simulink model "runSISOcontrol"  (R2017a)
settings: Solver=VariableStepAuto  StartTime=0.0  StopTime=12  RelTol=1e-3
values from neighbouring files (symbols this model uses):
  baud = 250000    [MISOcontrol.m]    (also in MISO_demo.m; runSteptest.m; SISOcontrol.m; init.m)
  com = 'COM4'    [MISOcontrol.m]    (also in MISO_demo.m; runSteptest.m; SISOcontrol.m; init.m)
  fixed_u1 = 0    [MISOcontrol.m]    (also in MISO_demo.m; SISOcontrol.m; init.m)
  fixed_u2 = 0    [MISOcontrol.m]    (also in MISO_demo.m; SISOcontrol.m; init.m)
  fixed_u3 = 0    [MISOcontrol.m]    (also in MISO_demo.m; SISOcontrol.m; init.m)
  fTf = 0.1    [MISOcontrol.m]    (also in MISO_demo.m; runSteptest.m; SISOcontrol.m; init.m)
  fTl = 0.05    [MISOcontrol.m]    (also in MISO_demo.m; runSteptest.m; SISOcontrol.m; init.m)
  fTt = 0.05    [MISOcontrol.m]    (also in MISO_demo.m; runSteptest.m; SISOcontrol.m; init.m)
  Kc = 1/k*tau1/(tauc+theta)    [SIMCPI.m]    (also in SIMCPI_nosat.m)
  step_d1 = -2.5    [MISOcontrol.m]    (also in MISO_demo.m; SISOcontrol.m = -2; init.m = 0)
  step_d2 = +2.5    (= 2.5)    [MISOcontrol.m]    (also in MISO_demo.m; SISOcontrol.m = 2; init.m = 0)
  step_ys1 = 5    [MISOcontrol.m]    (also in MISO_demo.m; SISOcontrol.m = 4)
  step_ys2 = -5    [MISOcontrol.m]    (also in MISO_demo.m; SISOcontrol.m = -4)
  stepTime1 = 30    [MISO_demo.m]    (also in SISOcontrol.m = 2)
  stepTime2 = 60    [MISO_demo.m]    (also in SISOcontrol.m = 4)
  stepTime_d1 = 90    [MISOcontrol.m]    (also in MISO_demo.m; SISOcontrol.m = 6; init.m = 0)
  stepTime_d2 = 120    [MISOcontrol.m]    (also in MISO_demo.m; SISOcontrol.m = 8; init.m = 0)
  tauI = min(tau1,4*(tauc+theta))    [SIMCPI.m]    (also in SIMCPI_nosat.m)
  Ts = 0.1    [identification.m]    (also in MISOcontrol.m; MISO_demo.m; runSteptest.m; SISOcontrol.m)
  turnOn_u1 = 1    [MISOcontrol.m]    (also in MISO_demo.m; SISOcontrol.m = 0)
  turnOn_u2 = 1    [MISOcontrol.m]    (also in MISO_demo.m; SISOcontrol.m = 0)
  turnOn_u3 = 0    [MISOcontrol.m]    (also in MISO_demo.m; SISOcontrol.m = 1)
  turnOn_y1 = 1    [MISOcontrol.m]    (also in MISO_demo.m; SISOcontrol.m = 0)
  turnOn_y2 = 0    [MISOcontrol.m]    (also in MISO_demo.m; SISOcontrol.m = 1)
  y0 = sb_T+3    (= 30)    [MISOcontrol.m]    (also in MISO_demo.m = sb_T; SISOcontrol.m = 0; init.m = 0; MIMOcontrol.m = 27)
  y_s0 = 0    [MISOcontrol.m]    (also in MISO_demo.m; SISOcontrol.m = 4)
undefined symbols (not defined in the file or in its folder): Kb
libraries: simulink x1, tom_lib x1

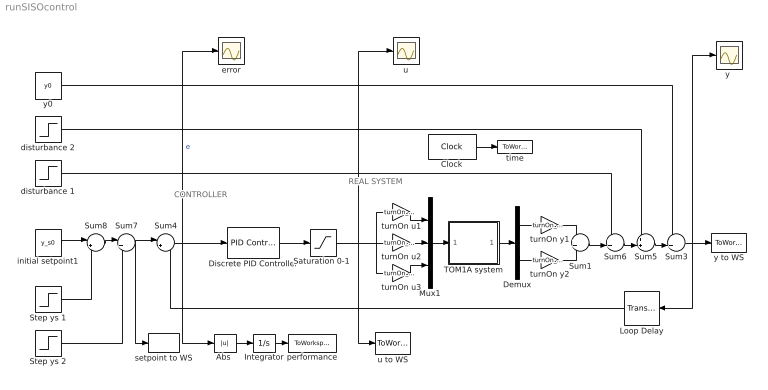
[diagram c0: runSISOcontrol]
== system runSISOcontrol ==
  note: CONTROLLER
  note: REAL SYSTEM
  "Abs " : Abs  ZeroCross=off
  Clock : Clock
  Demux : Demux  Outputs=2
  Discrete PID Controller : simulink/Continuous/PID Controller  Controller=PI  TimeDomain=Discrete-time  SampleTime=Ts  IntegratorMethod=Forward Euler  FilterMethod=Forward Euler  Form=Parallel  UseFilter=on  ControllerParametersSource=internal  P=Kc  I=Kc/tauI  D=0  N=100  InitialConditionSource=internal  InitialConditionForIntegrator=0  InitialConditionForFilter=0  ExternalReset=none  ZeroCross=off  LimitOutput=on  UpperSaturationLimit=1  LowerSaturationLimit=0  LinearizeAsGain=off  AntiWindupMode=clamping  Kb=Kb  TrackingMode=off  Kt=1  PParamMin=[]  PParamMax=[]  IParamMin=[]  IParamMax=[]  DParamMin=[]  DParamMax=[]  NParamMin=[]  NParamMax=[]  KbParamMin=[]  KbParamMax=[]  KtParamMin=[]  KtParamMax=[]  POutMin=[]  POutMax=[]  IOutMin=[]  IOutMax=[]  DOutMin=[]  DOutMax=[]  NOutMin=[]  NOutMax=[]  KbOutMin=[]  KbOutMax=[]  KtOutMin=[]  KtOutMax=[]  IntegratorOutMin=[]  IntegratorOutMax=[]  FilterOutMin=[]  FilterOutMax=[]  SumOutMin=[]  SumOutMax=[]  SumI1OutMin=[]  SumI1OutMax=[]  SumI2OutMin=[]  SumI2OutMax=[]  SumI3OutMin=[]  SumI3OutMax=[]  SumDOutMin=[]  SumDOutMax=[]  SaturationOutMin=[]  SaturationOutMax=[]  IntegratorContinuousStateAttributes=''  IntegratorStateMustResolveToSignalObject=off  IntegratorRTWStateStorageClass=Auto  FilterContinuousStateAttributes=''  FilterStateMustResolveToSignalObject=off  FilterRTWStateStorageClass=Auto  DifferentiatorICPrevScaledInput=0  DifferentiatorOutMin=[]  DifferentiatorOutMax=[]  InitialConditionSetting=State (most efficient)
  Integrator : Integrator  ZeroCross=off
  Loop Delay : TransportDelay  DelayTime=0.1
  Mux1 : Mux  Inputs=3
  "Saturation 0-1 " : Saturate  UpperLimit=1  LowerLimit=0  ZeroCross=off
  Step ys 1 : Step  Time=stepTime1  After=step_ys1  SampleTime=Ts  ZeroCross=off
  Step ys 2 : Step  Time=stepTime2  After=step_ys2  SampleTime=Ts  ZeroCross=off
  Sum1 : Sum
  Sum3 : Sum  Inputs=-+|
  Sum4 : Sum  Inputs=|+-
  Sum5 : Sum  Inputs=++|
  Sum6 : Sum  Inputs=++|
  Sum7 : Sum  Inputs=|++
  Sum8 : Sum  Inputs=|++
  TOM1A system : Subsystem
  disturbance 1 : Step  Time=stepTime_d1  After=step_d1  SampleTime=Ts  ZeroCross=off
  disturbance 2 : Step  Time=stepTime_d2  After=step_d2  SampleTime=Ts  ZeroCross=off
  error : Scope
  initial setpoint1 : Constant  Value=y_s0  SampleTime=Ts
  performance : ToWorkspace  VariableName=IAE  SampleTime=Ts
  setpoint to WS : ToWorkspace  VariableName=ys  SampleTime=Ts
  time : ToWorkspace  VariableName=time  SampleTime=Ts
  turnOn u1 : Gain  Gain=turnOn_u1
  turnOn u2 : Gain  Gain=turnOn_u2
  turnOn u3 : Gain  Gain=turnOn_u3
  turnOn y1 : Gain  Gain=turnOn_y1
  turnOn y2 : Gain  Gain=turnOn_y2
  u : Scope
  u to WS : ToWorkspace  VariableName=u  SampleTime=-1
  "y " : Scope
  y to WS : ToWorkspace  VariableName=y  SampleTime=Ts
  y0 : Constant  Value=y0
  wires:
  Clock/1 -> time/1
  "Saturation 0-1 "/1 -> u/1, turnOn u3/1, turnOn u1/1, turnOn u2/1, u to WS/1
  disturbance 1/1 -> Sum6/1
  Sum3/1 -> y to WS/1, "y "/1, Loop Delay/1
  Sum7/1 -> setpoint to WS/1, Sum4/1
  "Abs "/1 -> Integrator/1
  TOM1A system/1(y) -> Demux/1
  Sum4/1 -> Discrete PID Controller/1, "Abs "/1, error/1  "e"
  Integrator/1 -> performance/1
  Mux1/1 -> TOM1A system/1(u)
  turnOn u1/1 -> Mux1/1
  turnOn u2/1 -> Mux1/2
  turnOn u3/1 -> Mux1/3
  Demux/1 -> turnOn y1/1
  Demux/2 -> turnOn y2/1
  turnOn y2/1 -> Sum1/2
  turnOn y1/1 -> Sum1/1
  Discrete PID Controller/1 -> "Saturation 0-1 "/1
  Loop Delay/1 -> Sum4/2
  Sum1/1 -> Sum6/2
  Sum6/1 -> Sum5/2
  disturbance 2/1 -> Sum5/1
  Sum5/1 -> Sum3/2
  y0/1 -> Sum3/1
  Step ys 2/1 -> Sum7/2
  Sum8/1 -> Sum7/1
  initial setpoint1/1 -> Sum8/1
  Step ys 1/1 -> Sum8/2

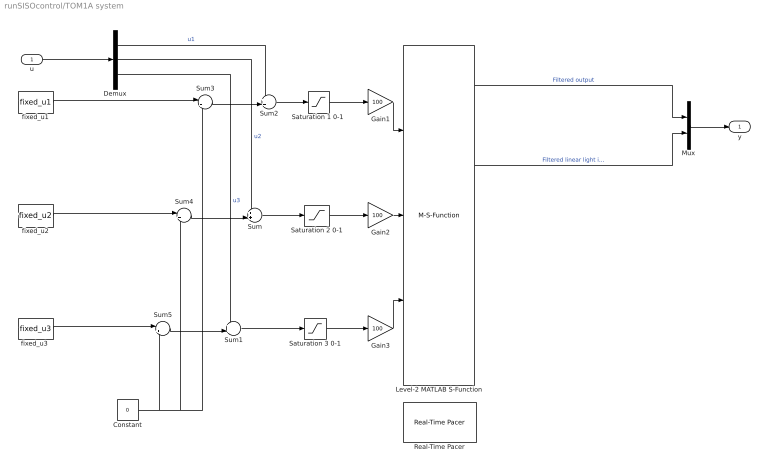
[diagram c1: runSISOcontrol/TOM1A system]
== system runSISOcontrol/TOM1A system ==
  u : Inport
  Constant : Constant  Value=0
  Demux : Demux  Outputs=3
  Gain1 : Gain  Gain=100
  Gain2 : Gain  Gain=100
  Gain3 : Gain  Gain=100
  Level-2 MATLAB S-Function : M-S-Function  FunctionName=tom1ar8  Parameters=Ts,com,baud,fTt,fTl,fTf
  Mux : Mux  Inputs=2
  Real-Time Pacer : tom_lib/Real-Time Pacer  simTimePerRealTime=1
  "Saturation 1 0-1 " : Saturate  UpperLimit=1  LowerLimit=0  ZeroCross=off
  Saturation 2 0-1 : Saturate  UpperLimit=1  LowerLimit=0  ZeroCross=off
  Saturation 3 0-1 : Saturate  UpperLimit=1  LowerLimit=0  ZeroCross=off
  Sum : Sum  Inputs=++|
  Sum1 : Sum  Inputs=++|
  Sum2 : Sum  Inputs=++|
  Sum3 : Sum  Inputs=|++
  Sum4 : Sum  Inputs=|++
  Sum5 : Sum  Inputs=|++
  fixed_u1 : Constant  Value=fixed_u1
  fixed_u2 : Constant  Value=fixed_u2
  "fixed_u3 " : Constant  Value=fixed_u3
  y : Outport
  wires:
  Level-2 MATLAB S-Function/14 -> ?  "Fan filtered  rpm"
  Level-2 MATLAB S-Function/3 -> ?  "Derivative of internal temperature"
  Level-2 MATLAB S-Function/4 -> ?  "Filtered external temperature"
  Level-2 MATLAB S-Function/13 -> ?  "Fan voltage"
  Level-2 MATLAB S-Function/11 -> ?  "Bulb voltage"
  Level-2 MATLAB S-Function/8 -> ?  "Filtered logaritmic light intensity"
  Level-2 MATLAB S-Function/1 -> ?  "Board temperature"
  Level-2 MATLAB S-Function/5 -> ?  "Derivate of external temperature"
  Level-2 MATLAB S-Function/12 -> ?  "Fan current"
  Level-2 MATLAB S-Function/9 -> ?  "Derivate of logaritmic light intensity"
  Level-2 MATLAB S-Function/16 -> ?  "Count of fan rpm"
  Level-2 MATLAB S-Function/15 -> ?  "Derivate of fan rpm"
  Level-2 MATLAB S-Function/10 -> ?  "Bulb current"
  Level-2 MATLAB S-Function/6 -> Mux/2  "Filtered linear light intensity"
  Level-2 MATLAB S-Function/7 -> ?  "Derivate of linear light intensity"
  Demux/1 -> Sum2/1  "u1"
  Demux/2 -> Sum/1  "u2"
  Demux/3 -> Sum1/1  "u3"
  u/1 -> Demux/1
  Level-2 MATLAB S-Function/2 -> Mux/1  "Filtered output"
  Mux/1 -> y/1
  fixed_u1/1 -> Sum3/1
  Sum3/1 -> Sum2/2
  Constant/1 -> Sum5/2, Sum4/2, Sum3/2
  fixed_u2/1 -> Sum4/1
  "fixed_u3 "/1 -> Sum5/1
  Sum5/1 -> Sum1/2
  Sum4/1 -> Sum/2
  Gain1/1 -> Level-2 MATLAB S-Function/1
  Gain2/1 -> Level-2 MATLAB S-Function/2
  Gain3/1 -> Level-2 MATLAB S-Function/3
  Saturation 2 0-1/1 -> Gain2/1
  Sum/1 -> Saturation 2 0-1/1
  "Saturation 1 0-1 "/1 -> Gain1/1
  Sum2/1 -> "Saturation 1 0-1 "/1
  Saturation 3 0-1/1 -> Gain3/1
  Sum1/1 -> Saturation 3 0-1/1
